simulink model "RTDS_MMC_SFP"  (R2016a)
settings: Solver=FixedStepAuto  StartTime=0.0  StopTime=0.4  RelTol=1e-3
PreLoadFcn:
  | % --- DO NOT REMOVE THIS CODE (2024.3.b1) ---
  |     % create Simulink variants
  |     if not(exist('variant_simulation', 'var'))
  |         variant_simulation = Simulink.Variant('SIMULINK_MODE==0');
  |     end
  |     if not(exist('variant_generation', 'var'))
  |         variant_generation = Simulink.Variant('SIMULINK_MODE==1');
  |     end
  | 
  |     % check SDK version
  |     required_lib_version = 3900.3;
  |     required_lib_ver_str = '2024.3';
  |     lib_path = [getenv('IX_SIMULINK_ACG_BB_3') '\simulink\blocks\BoomBox.slx'];
  |     if exist(lib_path, 'file')
  |         lib_version = str2double(Simulink.MDLInfo(lib_path).ModelVersion); % fullpath to avoid getting shadowing files
  |         if lib_version < required_lib_version || isnan(lib_version)
  |             error(['The model ''' bdroot ''' has been saved with a more recent version of ACG SDK (' required_lib_ver_str ') and might not work as expected. <a href="matlab:private_end_string = ''--- PLACE YOUR CODE BELOW THIS LINE ---'';private_fcn = get_param(bdroot, ''PreLoadFcn'');private_end_index = strfind(private_fcn, private_end_string);set_param(bdroot, ''PreLoadFcn'', strtrim(private_fcn(private_end_index(end)+length(private_end_string):end)));private_fcn = get_param(bdroot, ''PostLoadFcn'');private_end_index = strfind(private_fcn, private_end_string);set_param(bdroot, ''PostLoadFcn'', strtrim(private_fcn(private_end_index(end)+length(private_end_string):end)));private_fcn = get_param(bdroot, ''InitFcn'');private_end_index = strfind(private_fcn, private_end_string);set_param(bdroot, ''InitFcn'', strtrim(private_fcn(private_end_index(end)+length(private_end_string):end)));clear private_end_string private_fcn private_end_index;open(bdroot);">Click here</a> to continue anyway, or download the latest version of the SDK at <a href="www.imperix.com/downloads">www.imperix.ch/downloads</a>.']);
  |         end
  |     elseif exist(getenv('IX_SIMULINK_ACG_BB_3'), 'dir')
  |         error(['Library file for imperix ACG SDK not found in path ''' lib_path '''. Please try to re-install ACG SDK (<a href="www.imperix.com/downloads">www.imperix.ch/downloads</a>).']);
  |     else
  |         error('ACG SDK is not installed on this computer and the model will not work as expected. Please download ACG SDK at <a href="www.imperix.com/downloads">www.imperix.ch/downloads</a>, install it, and reopen the model.');
  |     end
  |     clear required_lib_version required_lib_ver_str lib_path lib_version;
  | 
  |     ix_acg_path = getenv('IX_SIMULINK_ACG_BB_3');
  |     addpath(fullfile(ix_acg_path, 'simulink\target'));
  |     addpath(fullfile(ix_acg_path, 'simulink\blocks'));
  |     addpath(fullfile(ix_acg_path, 'simulink\functions'));
  |     sl_refresh_customizations;
  |     clear ix_acg_path;
  | 
  |     % The SIMULINK_MODE variable is created in the base
  |     % workspace in the PostLoadFcn from the block whose id is kb0101
  |     % All opened models share a common variant configuration.
  | 
  |     Model_PreLoadFcn(bdroot);
  | % --- PLACE YOUR CODE BELOW THIS LINE ---
PostLoadFcn:
  | % --- DO NOT REMOVE THIS CODE (2024.3.b1) ---
  |     % change the execution mode of simulink depending on the radio button:
  |     if(strcmp('Automated Code Generation',get_param(Find_imperix_blocks(bdroot,'Configuration'),'SLMODE')))
  |         assignin('base', 'SIMULINK_MODE', 1);
  |     else
  |         assignin('base', 'SIMULINK_MODE', 0);
  |     end
  | 
  |     Model_PostLoadFcn(bdroot);
  | % --- PLACE YOUR CODE BELOW THIS LINE ---
InitFcn:
  | % --- DO NOT REMOVE THIS CODE (2024.3.b1) ---
  |     % check SDK version
  |     required_lib_version = 3900.3;
  |     required_lib_ver_str = '2024.3';
  |     lib_path = [getenv('IX_SIMULINK_ACG_BB_3') '\simulink\blocks\BoomBox.slx'];
  |     if exist(lib_path, 'file')
  |         lib_version = str2double(Simulink.MDLInfo(lib_path).ModelVersion); % fullpath to avoid getting shadowing files
  |         if lib_version < required_lib_version || isnan(lib_version)
  |             error(['The model ''' bdroot ''' has been saved with a more recent version of ACG SDK (' required_lib_ver_str ') and might not work as expected. <a href="matlab:private_end_string = ''--- PLACE YOUR CODE BELOW THIS LINE ---'';private_fcn = get_param(bdroot, ''PreLoadFcn'');private_end_index = strfind(private_fcn, private_end_string);set_param(bdroot, ''PreLoadFcn'', strtrim(private_fcn(private_end_index(end)+length(private_end_string):end)));private_fcn = get_param(bdroot, ''PostLoadFcn'');private_end_index = strfind(private_fcn, private_end_string);set_param(bdroot, ''PostLoadFcn'', strtrim(private_fcn(private_end_index(end)+length(private_end_string):end)));private_fcn = get_param(bdroot, ''InitFcn'');private_end_index = strfind(private_fcn, private_end_string);set_param(bdroot, ''InitFcn'', strtrim(private_fcn(private_end_index(end)+length(private_end_string):end)));clear private_end_string private_fcn private_end_index;open(bdroot);">Click here</a> to continue anyway, or download the latest version of the SDK at <a href="www.imperix.com/downloads">www.imperix.ch/downloads</a>.']);
  |         end
  |     elseif exist(getenv('IX_SIMULINK_ACG_BB_3'), 'dir')
  |         error(['Library file for imperix ACG SDK not found in path ''' lib_path '''. Please try to re-install ACG SDK (<a href="www.imperix.com/downloads">www.imperix.ch/downloads</a>).']);
  |     else
  |         error('ACG SDK is not installed on this computer and the model will not work as expected. Please download ACG SDK at <a href="www.imperix.com/downloads">www.imperix.ch/downloads</a>, install it, and reopen the model.');
  |     end
  |     clear required_lib_version required_lib_ver_str lib_path lib_version;
  | 
  |     Model_InitFcn(bdroot);
  | % --- PLACE YOUR CODE BELOW THIS LINE ---
model workspace (MAT data in the model file):
  CTRLPERIOD = 0.0002
  TSAMPLE = 2e-06
  global_CLK_number = 0
  global_INT_number = 1
  global_SVM_instance_id = 0
  global_can_baud_rate = '1000000'
  global_comp_time = 0.2
  global_cycle_delay = 8e-05
  global_ip_addresses : cell (value not decoded)
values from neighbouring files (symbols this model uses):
  Ki_Vleg = 1/Ti    (= 2.95256991686)    [RTDS_MMC_SFP_init.m]
  Kp_Vleg = Tn/Ti    (= 0.14880952381)    [RTDS_MMC_SFP_init.m]
  N = 4    [RTDS_MMC_SFP_init.m]
  scale_factor = 0.5^16    (= 1.52587890625e-05)    [RTDS_MMC_SFP_init.m]
  Tsw = 1/fsw    (= 0.0008)    [RTDS_MMC_SFP_init.m]
  Vsm_max = 250    [RTDS_MMC_SFP_init.m]
undefined symbols (not defined in the file or in its folder): B, Board, Box, channel, DT, lane, Micro, ns, PRO, RCP, TPI, Vf
libraries: BoomBox x183, simulink x55
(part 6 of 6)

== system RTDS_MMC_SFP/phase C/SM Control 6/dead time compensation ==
  sign : Inport
  Vdc : Inport  Port=2
  m : Inport  Port=3
  Constant1 : Constant  Value=Vf  OutDataTypeStr=single
  Constant2 : Constant  Value=DT/Tsw  OutDataTypeStr=single
  Gain : Gain  Gain=0.5
  Product : Product
  Product1 : Product
  Product2 : Product
  Product3 : Product  Inputs=/*
  Sum : Sum  Inputs=|++
  Sum1 : Sum  Inputs=|++
  Sum2 : Sum  Inputs=|++
  m' : Outport
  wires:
  Gain/1 -> Product3/2
  Vdc/1 -> Product3/1, Sum1/1
  Product3/1 -> Sum/2
  Product2/1 -> Gain/1
  sign/1 -> Product2/2
  Sum2/1 -> Product2/1
  Product1/1 -> Sum2/2
  Product/1 -> Sum2/1
  Constant2/1 -> Product/2
  Sum1/1 -> Product/1
  Constant1/1 -> Product1/2, Sum1/2
  Sum/1 -> m'/1
  m/1 -> Sum/1, Product1/1

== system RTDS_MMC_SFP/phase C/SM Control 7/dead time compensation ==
  sign : Inport
  Vdc : Inport  Port=2
  m : Inport  Port=3
  Constant1 : Constant  Value=Vf  OutDataTypeStr=single
  Constant2 : Constant  Value=DT/Tsw  OutDataTypeStr=single
  Gain : Gain  Gain=0.5
  Product : Product
  Product1 : Product
  Product2 : Product
  Product3 : Product  Inputs=/*
  Sum : Sum  Inputs=|++
  Sum1 : Sum  Inputs=|++
  Sum2 : Sum  Inputs=|++
  m' : Outport
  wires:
  m/1 -> Product1/1, Sum/1
  Sum/1 -> m'/1
  Constant1/1 -> Sum1/2, Product1/2
  Sum1/1 -> Product/1
  Constant2/1 -> Product/2
  Product/1 -> Sum2/1
  Product1/1 -> Sum2/2
  Sum2/1 -> Product2/1
  sign/1 -> Product2/2
  Product2/1 -> Gain/1
  Product3/1 -> Sum/2
  Vdc/1 -> Sum1/1, Product3/1
  Gain/1 -> Product3/2

== matlab function RTDS_MMC_SFP/Vertical arm
voltages balancing/MATLAB Function ==
function y = fcn(u, theta)
M= [cos(theta)                  -1/sqrt(3)*sin(theta)           1/sqrt(3)*sin(theta);
    1/sqrt(3)*sin(theta-2*pi/3) cos(theta-2*pi/3)               -1/sqrt(3)*sin(theta-2*pi/3);
    -1/sqrt(3)*sin(theta+2*pi/3) 1/sqrt(3)*sin(theta+2*pi/3)    cos(theta+2*pi/3)];
y = M*u;

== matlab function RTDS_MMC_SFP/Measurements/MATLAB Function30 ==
function y = sbi2int32(u1,u2)
  y = int32(0); % fix simulink bug: force compiled size of output
  y = typecast([uint16(u1) uint16(u2)], 'int32');

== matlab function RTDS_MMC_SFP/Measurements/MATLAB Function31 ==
function y = sbi2int32(u1,u2)
  y = int32(0); % fix simulink bug: force compiled size of output
  y = typecast([uint16(u1) uint16(u2)], 'int32');

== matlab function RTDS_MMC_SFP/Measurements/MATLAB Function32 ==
function y = sbi2int32(u1,u2)
  y = int32(0); % fix simulink bug: force compiled size of output
  y = typecast([uint16(u1) uint16(u2)], 'int32');

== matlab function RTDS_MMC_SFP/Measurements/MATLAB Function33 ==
function y = sbi2int32(u1,u2)
  y = int32(0); % fix simulink bug: force compiled size of output
  y = typecast([uint16(u1) uint16(u2)], 'int32');

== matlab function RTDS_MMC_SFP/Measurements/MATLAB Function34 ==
function y = sbi2int32(u1,u2)
  y = int32(0); % fix simulink bug: force compiled size of output
  y = typecast([uint16(u1) uint16(u2)], 'int32');

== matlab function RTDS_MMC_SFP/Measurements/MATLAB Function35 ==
function y = sbi2int32(u1,u2)
  y = int32(0); % fix simulink bug: force compiled size of output
  y = typecast([uint16(u1) uint16(u2)], 'int32');

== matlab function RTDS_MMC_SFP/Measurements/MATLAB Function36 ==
function y = sbi2int32(u1,u2)
  y = int32(0); % fix simulink bug: force compiled size of output
  y = typecast([uint16(u1) uint16(u2)], 'int32');

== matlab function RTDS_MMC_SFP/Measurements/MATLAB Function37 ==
function y = sbi2int32(u1,u2)
  y = int32(0); % fix simulink bug: force compiled size of output
  y = typecast([uint16(u1) uint16(u2)], 'int32');

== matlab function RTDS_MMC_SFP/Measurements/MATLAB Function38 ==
function y = sbi2int32(u1,u2)
  y = int32(0); % fix simulink bug: force compiled size of output
  y = typecast([uint16(u1) uint16(u2)], 'int32');

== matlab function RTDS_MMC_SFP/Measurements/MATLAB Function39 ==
function y = sbi2int32(u1,u2)
  y = int32(0); % fix simulink bug: force compiled size of output
  y = typecast([uint16(u1) uint16(u2)], 'int32');

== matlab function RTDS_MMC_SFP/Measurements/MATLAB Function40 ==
function y = sbi2int32(u1,u2)
  y = int32(0); % fix simulink bug: force compiled size of output
  y = typecast([uint16(u1) uint16(u2)], 'int32');

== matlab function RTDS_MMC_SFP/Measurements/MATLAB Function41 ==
function y = sbi2int32(u1,u2)
  y = int32(0); % fix simulink bug: force compiled size of output
  y = typecast([uint16(u1) uint16(u2)], 'int32');

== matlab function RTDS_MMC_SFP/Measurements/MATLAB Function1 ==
function y = sbi2int32(u1,u2)
  y = int32(0); % fix simulink bug: force compiled size of output
  y = typecast([uint16(u1) uint16(u2)], 'int32');

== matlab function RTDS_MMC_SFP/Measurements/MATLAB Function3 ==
function y = sbi2int32(u1,u2)
  y = int32(0); % fix simulink bug: force compiled size of output
  y = typecast([uint16(u1) uint16(u2)], 'int32');

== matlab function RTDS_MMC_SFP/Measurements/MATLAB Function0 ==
function y = sbi2int32(u1,u2)
  y = int32(0); % fix simulink bug: force compiled size of output
  y = typecast([uint16(u1) uint16(u2)], 'int32');

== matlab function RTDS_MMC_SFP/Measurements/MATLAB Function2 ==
function y = sbi2int32(u1,u2)
  y = int32(0); % fix simulink bug: force compiled size of output
  y = typecast([uint16(u1) uint16(u2)], 'int32');

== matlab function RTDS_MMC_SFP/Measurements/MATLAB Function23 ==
function y = sbi2int32(u1,u2)
  y = int32(0); % fix simulink bug: force compiled size of output
  y = typecast([uint16(u1) uint16(u2)], 'int32');

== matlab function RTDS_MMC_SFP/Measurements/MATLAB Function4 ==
function y = sbi2int32(u1,u2)
  y = int32(0); % fix simulink bug: force compiled size of output
  y = typecast([uint16(u1) uint16(u2)], 'int32');

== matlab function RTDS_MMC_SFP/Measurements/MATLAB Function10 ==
function y = sbi2int32(u1,u2)
  y = int32(0); % fix simulink bug: force compiled size of output
  y = typecast([uint16(u1) uint16(u2)], 'int32');

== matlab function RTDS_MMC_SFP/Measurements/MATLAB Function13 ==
function y = sbi2int32(u1,u2)
  y = int32(0); % fix simulink bug: force compiled size of output
  y = typecast([uint16(u1) uint16(u2)], 'int32');

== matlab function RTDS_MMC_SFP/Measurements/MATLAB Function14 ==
function y = sbi2int32(u1,u2)
  y = int32(0); % fix simulink bug: force compiled size of output
  y = typecast([uint16(u1) uint16(u2)], 'int32');

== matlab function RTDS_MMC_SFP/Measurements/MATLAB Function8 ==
function y = sbi2int32(u1,u2)
  y = int32(0); % fix simulink bug: force compiled size of output
  y = typecast([uint16(u1) uint16(u2)], 'int32');

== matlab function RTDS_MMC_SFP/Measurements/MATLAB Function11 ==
function y = sbi2int32(u1,u2)
  y = int32(0); % fix simulink bug: force compiled size of output
  y = typecast([uint16(u1) uint16(u2)], 'int32');

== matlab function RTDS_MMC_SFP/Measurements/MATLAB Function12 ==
function y = sbi2int32(u1,u2)
  y = int32(0); % fix simulink bug: force compiled size of output
  y = typecast([uint16(u1) uint16(u2)], 'int32');

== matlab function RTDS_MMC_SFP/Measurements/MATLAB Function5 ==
function y = sbi2int32(u1,u2)
  y = int32(0); % fix simulink bug: force compiled size of output
  y = typecast([uint16(u1) uint16(u2)], 'int32');

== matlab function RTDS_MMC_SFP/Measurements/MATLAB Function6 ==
function y = sbi2int32(u1,u2)
  y = int32(0); % fix simulink bug: force compiled size of output
  y = typecast([uint16(u1) uint16(u2)], 'int32');

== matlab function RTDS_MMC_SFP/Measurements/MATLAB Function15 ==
function y = sbi2int32(u1,u2)
  y = int32(0); % fix simulink bug: force compiled size of output
  y = typecast([uint16(u1) uint16(u2)], 'int32');

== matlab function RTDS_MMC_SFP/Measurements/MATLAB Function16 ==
function y = sbi2int32(u1,u2)
  y = int32(0); % fix simulink bug: force compiled size of output
  y = typecast([uint16(u1) uint16(u2)], 'int32');

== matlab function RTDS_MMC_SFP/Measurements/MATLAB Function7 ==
function y = sbi2int32(u1,u2)
  y = int32(0); % fix simulink bug: force compiled size of output
  y = typecast([uint16(u1) uint16(u2)], 'int32');

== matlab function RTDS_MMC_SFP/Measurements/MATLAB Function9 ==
function y = sbi2int32(u1,u2)
  y = int32(0); % fix simulink bug: force compiled size of output
  y = typecast([uint16(u1) uint16(u2)], 'int32');

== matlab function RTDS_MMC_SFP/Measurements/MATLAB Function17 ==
function y = sbi2int32(u1,u2)
  y = int32(0); % fix simulink bug: force compiled size of output
  y = typecast([uint16(u1) uint16(u2)], 'int32');

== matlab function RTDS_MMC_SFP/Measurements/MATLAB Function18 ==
function y = sbi2int32(u1,u2)
  y = int32(0); % fix simulink bug: force compiled size of output
  y = typecast([uint16(u1) uint16(u2)], 'int32');

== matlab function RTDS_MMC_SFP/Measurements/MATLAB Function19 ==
function y = sbi2int32(u1,u2)
  y = int32(0); % fix simulink bug: force compiled size of output
  y = typecast([uint16(u1) uint16(u2)], 'int32');

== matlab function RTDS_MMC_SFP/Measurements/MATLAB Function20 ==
function y = sbi2int32(u1,u2)
  y = int32(0); % fix simulink bug: force compiled size of output
  y = typecast([uint16(u1) uint16(u2)], 'int32');

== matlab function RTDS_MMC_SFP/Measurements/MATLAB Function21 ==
function y = sbi2int32(u1,u2)
  y = int32(0); % fix simulink bug: force compiled size of output
  y = typecast([uint16(u1) uint16(u2)], 'int32');

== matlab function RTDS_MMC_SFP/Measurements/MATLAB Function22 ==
function y = sbi2int32(u1,u2)
  y = int32(0); % fix simulink bug: force compiled size of output
  y = typecast([uint16(u1) uint16(u2)], 'int32');

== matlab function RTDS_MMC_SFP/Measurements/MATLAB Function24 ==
function y = sbi2int32(u1,u2)
  y = int32(0); % fix simulink bug: force compiled size of output
  y = typecast([uint16(u1) uint16(u2)], 'int32');

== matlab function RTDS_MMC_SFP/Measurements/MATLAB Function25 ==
function y = sbi2int32(u1,u2)
  y = int32(0); % fix simulink bug: force compiled size of output
  y = typecast([uint16(u1) uint16(u2)], 'int32');

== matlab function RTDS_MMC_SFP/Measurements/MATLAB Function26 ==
function y = sbi2int32(u1,u2)
  y = int32(0); % fix simulink bug: force compiled size of output
  y = typecast([uint16(u1) uint16(u2)], 'int32');

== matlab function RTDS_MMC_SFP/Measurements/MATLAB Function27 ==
function y = sbi2int32(u1,u2)
  y = int32(0); % fix simulink bug: force compiled size of output
  y = typecast([uint16(u1) uint16(u2)], 'int32');

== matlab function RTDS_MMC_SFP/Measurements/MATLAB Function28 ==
function y = sbi2int32(u1,u2)
  y = int32(0); % fix simulink bug: force compiled size of output
  y = typecast([uint16(u1) uint16(u2)], 'int32');

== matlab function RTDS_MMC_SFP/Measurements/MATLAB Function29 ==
function y = sbi2int32(u1,u2)
  y = int32(0); % fix simulink bug: force compiled size of output
  y = typecast([uint16(u1) uint16(u2)], 'int32');
